TYPE ACS_DRIVE_TYPE :
STRUCT
	//Synchronization Variable (Read/Write Routines)
	_InputCurrentPosition AT %I* 		: REAL;
	//Synchronization Variable (Read/Write Routines)
	_InputStatus AT %I* 					: BITARR32;
	//Synchronization Variable (Read/Write Routines)
	_InputFaults AT %I* 					: BITARR32;
	//Synchronization Variable (Read/Write Routines)
	_InputDigitalInputs AT %I* 			: BITARR32;
	//Synchronization Variable (Read/Write Routines)
	_InputDigitalOutputs AT %I* 			: BITARR32;
	//Synchronization Variable (Read/Write Routines)
	_InputAnalogOutput AT %I* 			: REAL;
	//Synchronization Variable (Read/Write Routines)
	_InputAnalogInput AT %I* 			: REAL;
	
	//Synchronization Variable (Read/Write Routines)
	_OutputCommand AT %Q* 				: USINT;
	//Synchronization Variable (Read/Write Routines)
	_OutputMoveSelect AT %Q* 			: USINT;
	//Synchronization Variable (Read/Write Routines)
	_OutputTargetPosition AT %Q* 		: REAL;
	//Synchronization Variable (Read/Write Routines)
	_OutputTargetVelocity AT %Q* 		: REAL;
	//Synchronization Variable (Read/Write Routines)
	_OutputTargetAcceleration AT %Q* 	: REAL;
	//Synchronization Variable (Read/Write Routines)
	_OutputTargetDeceleration AT %Q* 	: REAL;
	//Synchronization Variable (Read/Write Routines)
	_OutputTargetForce AT %Q* 			: REAL;
	//Synchronization Variable (Read/Write Routines)
	_OutputTargetMotionType AT %Q* 		: UDINT;
	//Synchronization Variable (Read/Write Routines)
	_OutputDigitalOutputs AT %Q* 		: BITARR32;	

	//User Command to write to drive
	OutputCommand				: USINT;
	//User indexed move select to write to drive
	OutputMoveSelect			: USINT;
	//User target position to write to drive in mm or rotary units
	OutputTargetPosition		: REAL;
	//User target velocity to write to drive in mm/s or rotary units
	OutputTargetVelocity 		: REAL;
	//User target acceleration to write to drive in mm/s/s or rotary units
	OutputTargetAcceleration	: REAL;
	//User target Deceleration to write to drive in mm/s/s or rotary units
	OutputTargetDeceleration	: REAL;
	//User target force to write to drive in % peak force
	OutputTargetForce			: REAL;
	//User target motion to write to drive
	OutputTargetMotionType 		: UDINT;
	
	//Assign digital output (must be configured as Not Assigned in TMI
	OutputDigitalOutput1		: BOOL;
	//Assign digital output (must be configured as Not Assigned in TMI
	OutputDigitalOutput2		:	BOOL;
	
	//User Current Position in mm or rotary units
	InputCurrentPosition 			: REAL;
	//User Access to Analog Output
	InputAnalogOutput				: REAL;
	//User Access to Analog Input
	InputAnalogInput 				: REAL;
	
	//Digital input read From Drive
	InputDigitalInput1					: BOOL;
	//Digital input read From Drive
	InputDigitalInput2					: BOOL;
	//Digital input read From Drive
	InputDigitalInput3					: BOOL;
	//Digital input read From Drive
	InputDigitalInput4					: BOOL;
	
	//Digital output read from drive
	InputDigitalOutput1					: BOOL;
	//Digital output read from drive
	InputDigitalOutput2					: BOOL;
	
	//Status bits from drive
	InputStatusDriveEnabled 			: BOOL;
	//Status bits from drive
	InputStatusDriveHomed 				: BOOL;
	//Status bits from drive
	InputStatusDriveInMotion 			: BOOL;
	//Status bits from drive
	InputStatusDriveSoftwareStop 		: BOOL;
	//Status bits from drive
	InputStatusDriveBrakeNotActive 		: BOOL;
	//Status bits from drive
	InputStatusDriveTMISoftwareControl 	: BOOL;
	
	//Active when there is any fault
	InputFaultActive					: BOOL;
	
	//Fault bits from drive
	InputFaultsDrivePositiveLimit 		: BOOL;
	//Fault bits from drive
	InputFaultsDriveNegativeLimit 		: BOOL;
	//Fault bits from drive
	InputFaultsDriveSoftwareStop 		: BOOL;
	//Fault bits from drive
	InputFaultsDrivePositionError 		: BOOL;
	//Fault bits from drive
	InputFaultsDriveFeedbackError 		: BOOL;
	//Fault bits from drive
	InputFaultsDriveOvercurrentError 	: BOOL;
	//Fault bits from drive
	InputFaultsDriveMotorOvertempError 	: BOOL;
	//Fault bits from drive
	InputFaultsDriveOvertempError 		: BOOL;
	//Fault bits from drive
	InputFaultsDriveOvervoltageError 	: BOOL;
	//Fault bits from drive
	InputFaultsDriveUndervoltageError 	: BOOL;
	//Fault bits from drive
	InputFaultsDriveFlashError 			: BOOL;
	//Fault bits from drive
	InputFaultsDriveI2TLimitError 		: BOOL;
	//Fault bits from drive
	InputFaultsDriveShortCircuitError 	: BOOL;
	//Fault bits from drive
	InputFaultsDriveWatchdogResetError 	: BOOL;
END_STRUCT
END_TYPE
